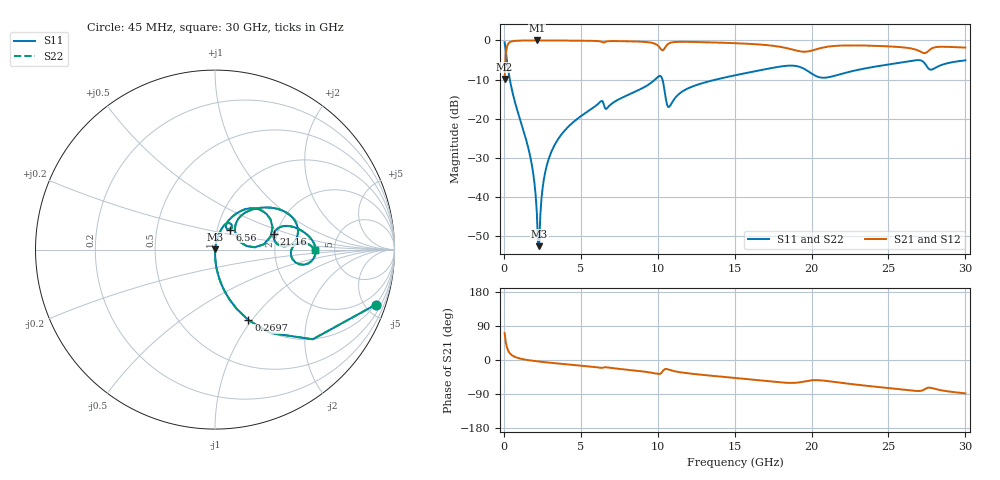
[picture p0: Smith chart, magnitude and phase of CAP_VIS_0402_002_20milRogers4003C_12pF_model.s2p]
! S-parameter model data by Modelithics Inc.  support@modelithics.com  813-866-6335  Tampa FL USA
! S-Parameter data specifications:
! Substrate: 20-mil Rogers 4003C, substrate thickness, H=0.508mm, Dielectric constant, Er=3.75
! PCB Mounting Pad Footprint: Pad width, PadW=0.50mm , Pad length, PadL=0.50mm , Pad gap, PadG (edge-to-edge)=0.40mm , Reference planes=1.4mm apart
! Created Wed Nov 18 12:51:33 2015
# hz S ma R 50
! 2 Port Network Data from SP1.SP block
! freq  magS11  angS11  magS21  angS21  magS12  angS12  magS22  angS22
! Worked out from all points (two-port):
!   401 points, 45 MHz to 30 GHz, reference 50 ohm
!   highest |S21| = -0.01 dB at 2.142 GHz (marker M1); lowest = -9.8 dB at 45 MHz (marker M2)
!   |S21| within 3 dB of the highest: 137.5 MHz to 27.15 GHz (27.02 GHz wide, 198 % of centre); 27.5 GHz to end of sweep
!   lowest |S11| = -52.6 dB at 2.292 GHz (marker M3), VSWR 1.00, Z = 50.2 + j0.179 ohm
!   |S11| at or under -10 dB: 385.7 MHz to 9.822 GHz (9.437 GHz wide, 185 % of centre); 10.31 GHz to 13.78 GHz (3.476 GHz wide, 28.9 % of centre)
!   |S22| runs from -52.6 to -0.5 dB; largest |S21 - S12| = 0
!   S11 on the Smith chart (normalised r, x): 45 MHz: 0.99, -5.84; 269.7 MHz: 0.99, -0.96; 6.56 GHz: 1.15, +0.26; 21.16 GHz: 1.93, +0.39; 30 GHz: 3.51, +0.00
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4.5e7  0.9465 -18.9  0.3227 71.1  0.3227 71.1  0.9465 -18.9
2.696625e8  0.4346 -64.7  0.9002 25.3  0.9002 25.3  0.4346 -64.7
6.441e8  0.185 -80.2  0.982 9.5  0.982 9.5  0.185 -80.2
1.767412e9  0.02893 -89.0  0.9983 -1.4  0.9983 -1.4  0.02893 -89.0
1.992075e9  0.01468 -87.5  0.9985 -2.7  0.9985 -2.7  0.01468 -87.5
2.14185e9  0.006218 -80.8  0.9986 -3.4  0.9986 -3.4  0.006218 -80.8
2.291625e9  0.002357 49.3  0.9985 -4.1  0.9985 -4.1  0.002357 49.3
2.666062e9  0.01992 79.8  0.9982 -5.8  0.9982 -5.8  0.01992 79.8
3.0405e9  0.03596 80.0  0.9976 -7.4  0.9976 -7.4  0.03596 80.0
5.062462e9  0.1098 73.6  0.9914 -15.2  0.9914 -15.2  0.1098 73.6
6.560212e9  0.1375 53.9  0.9508 -19.1  0.9508 -19.1  0.1375 53.9
9.0315e9  0.2474 57.7  0.9592 -30.1  0.9592 -30.1  0.2474 57.7
1.007992e10  0.3491 34.5  0.8328 -37.0  0.8328 -37.0  0.3491 34.5
1.075391e10  0.1421 34.1  0.9211 -25.9  0.9211 -25.9  0.1421 34.1
1.2027e10  0.247 52.0  0.9572 -35.4  0.9572 -35.4  0.247 52.0
1.50225e10  0.3585 40.8  0.9218 -47.4  0.9218 -47.4  0.3585 40.8
1.876688e10  0.4763 14.5  0.7635 -60.5  0.7635 -60.5  0.4763 14.5
2.003996e10  0.3732 3.0  0.7438 -53.5  0.7438 -53.5  0.3732 3.0
2.116328e10  0.3403 15.2  0.8372 -56.2  0.8372 -56.2  0.3403 15.2
2.505742e10  0.4949 12.2  0.8379 -74.2  0.8379 -74.2  0.4949 12.2
2.737894e10  0.5031 -9.6  0.6889 -76.6  0.6889 -76.6  0.5031 -9.6
3e10  0.5567 0.0  0.8101 -88.0  0.8101 -88.0  0.5567 0.0
